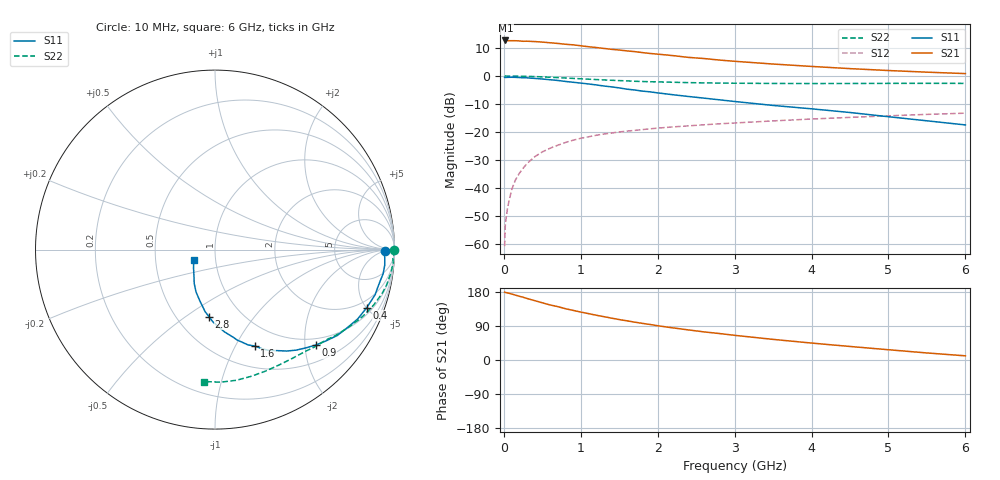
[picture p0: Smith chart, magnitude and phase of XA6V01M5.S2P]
! SIEMENS Discrete & RF Semiconductors
! BFY180
! Si NPN RF Bipolar Junction Transistor in MICRO-X
! VCE = 6 V  IC = 1.5 mA
! Common Emitter S-Parameters:  May  1997
# GHz  S  MA  R  50
!  f  S11  S21  S12  S22
! GHz  MAG  ANG  MAG  ANG  MAG  ANG  MAG  ANG
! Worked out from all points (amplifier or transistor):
!   36 points, 10 MHz to 6 GHz, reference 50 ohm
!   highest |S21| = 12.7 dB at 20 MHz (marker M1)
!   |S21| within 3 dB of that: start of sweep to 1.345 GHz
!   unconditionally stable (mu >= 1): 3.456 GHz to end of sweep
!   at 250 MHz: K = 0.09, MSG = 22.7 dB, |S12| = -33.0 dB
!   at 1.4 GHz: K = 0.57, MSG = 15.0 dB, |S12| = -20.4 dB
!   at 6 GHz: K = 1.06, MAG = 5.6 dB, |S12| = -13.3 dB
!   S11 on the Smith chart (normalised r, x): 10 MHz: 36, -5; 400 MHz: 1.41, -5.04; 900 MHz: 0.85, -2.23; 1.6 GHz: 0.74, -1.20; 2.8 GHz: 0.71, -0.62; 6 GHz: 0.78, -0.10
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0.01  0.9468 -0.4  4.286 178.9  0.0009 93.4  0.9979 -0.2
0.02  0.9415 -1.0  4.326 178.3  0.0023 84.0  0.9999 -0.6
0.05  0.947 -2.7  4.28 177.0  0.0045 85.1  0.9969 -1.5
0.1  0.9496 -5.2  4.282 174.2  0.0091 87.1  0.9925 -3.0
0.15  0.9464 -8.2  4.277 171.3  0.0137 85.1  0.9962 -4.4
0.25  0.9303 -13.3  4.183 165.7  0.0223 81.6  0.9897 -7.4
0.4  0.9055 -20.9  4.133 156.7  0.0358 76.0  0.9763 -11.6
0.6  0.8563 -30.5  3.933 145.3  0.0509 70.1  0.9494 -16.9
0.7  0.8324 -35.1  3.83 140.9  0.0576 66.9  0.9361 -19.3
0.8  0.7997 -39.6  3.702 135.4  0.0645 64.2  0.9207 -21.6
0.9  0.7728 -43.5  3.613 131.0  0.0709 61.5  0.906 -23.9
1.1  0.7204 -51.0  3.341 122.4  0.0816 57.3  0.8766 -27.8
1.4  0.6385 -61.7  3.002 110.5  0.0954 51.6  0.8384 -33.3
1.6  0.5811 -67.6  2.813 103.4  0.1032 48.7  0.8177 -36.5
2  0.4985 -78.3  2.461 90.4  0.1168 43.7  0.7847 -42.2
2.2  0.4617 -83.4  2.315 84.7  0.1227 41.5  0.7726 -45.1
2.6  0.4019 -91.8  2.054 74.2  0.1338 38.0  0.7534 -50.1
2.8  0.3749 -95.1  1.93 69.9  0.1394 36.5  0.7471 -52.6
3.5  0.2971 -106.6  1.637 54.4  0.1572 31.2  0.7351 -61.2
4.5  0.2221 -121.4  1.355 35.7  0.1818 24.0  0.7342 -74.0
5.5  0.1577 -139.3  1.171 18.6  0.2056 16.3  0.7393 -87.7
6  0.1331 -153.1  1.104 11.0  0.2161 12.2  0.7375 -94.6
